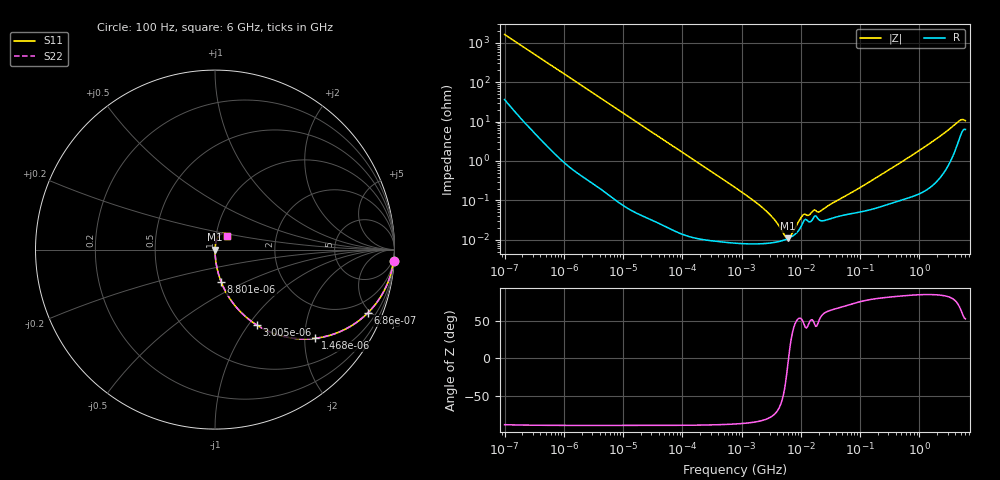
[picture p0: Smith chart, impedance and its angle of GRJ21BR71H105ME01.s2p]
!Murata Part Number: GRJ21BR71H105ME01
!These Parameters are Measured in Series Mode Connection
!Data Generated on Jun 19, 2026
!  o--ll--o
!Port1  Port2
!  o------o
!Operation Temp=25[degC], DC Bias Voltage=0[V]
!Freq. Start=100[Hz] Stop=6[GHz] 401[Steps]
# Hz S RI R 50
!Freq.(Hz) S11(Real) S11(Imag) S21(Real) S21(Imag) S12(Real) S12(Imag) S22(Real) S22(Imag)
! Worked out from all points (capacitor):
!   401 points, 100 Hz to 6 GHz, reference 50 ohm
!   read as one part in series: C = 972 nF near 109 Hz
!   lowest |Z| = 10.8 mohm at 6.075 MHz (marker M1)
!   series resonance near 6.209 MHz, so ESL is about 680 pH
!   S11 on the Smith chart (normalised r, x): 100 Hz: 2, -33; 686 Hz: 1.03, -4.80; 1.468 kHz: 1.01, -2.25; 3.005 kHz: 1.01, -1.10; 8.801 kHz: 1.00, -0.38; 6 GHz: 1.13, +0.17
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100  0.9949 -0.0608  0.00507 0.0608  0.00507 0.0608  0.9949 -0.0608
335  0.9583 -0.195  0.0417 0.195  0.0417 0.195  0.9583 -0.195
686  0.8505 -0.3533  0.1495 0.3533  0.1495 0.3533  0.8505 -0.3533
1468  0.5575 -0.4941  0.4425 0.4941  0.4425 0.4941  0.5575 -0.4941
2008  0.4035 -0.4881  0.5965 0.4881  0.5965 0.4881  0.4035 -0.4881
3005  0.2332 -0.4204  0.7668 0.4204  0.7668 0.4204  0.2332 -0.4204
4918  0.1029 -0.3014  0.8971 0.3014  0.8971 0.3014  0.1029 -0.3014
8801  0.035 -0.1815  0.965 0.1815  0.965 0.1815  0.035 -0.1815
40335  0.00196 -0.0411  0.998 0.0411  0.998 0.0411  0.00196 -0.0411
774597  8.63e-05 -0.00213  0.9999 0.00213  0.9999 0.00213  8.63e-05 -0.00213
2713602  8.13e-05 -0.000502  0.9999 0.000502  0.9999 0.000502  8.13e-05 -0.000502
3882480  8.74e-05 -0.000265  0.9999 0.000265  0.9999 0.000265  8.74e-05 -0.000265
5554849  0.000101 -6.12e-05  0.9999 6.12e-05  0.9999 6.12e-05  0.000101 -6.12e-05
6075234  0.000107 -1.19e-05  0.9999 1.19e-05  0.9999 1.19e-05  0.000107 -1.19e-05
6948629  0.000119 6.3e-05  0.9999 -6.3e-05  0.9999 -6.3e-05  0.000119 6.3e-05
1.039699e7  0.000237 0.000308  0.9998 -0.000308  0.9998 -0.000308  0.000237 0.000308
1.555665e7  0.000316 0.000404  0.9997 -0.000404  0.9997 -0.000404  0.000316 0.000404
2.128304e7  0.000308 0.000432  0.9997 -0.000432  0.9997 -0.000432  0.000308 0.000432
3.124326e8  0.000848 0.00599  0.9992 -0.00599  0.9992 -0.00599  0.000848 0.00599
1.565993e9  0.00303 0.0289  0.997 -0.0289  0.997 -0.0289  0.00303 0.0289
4.586474e9  0.0389 0.0892  0.9611 -0.0892  0.9611 -0.0892  0.0389 0.0892
6e9  0.0654 0.0741  0.9346 -0.0741  0.9346 -0.0741  0.0654 0.0741
